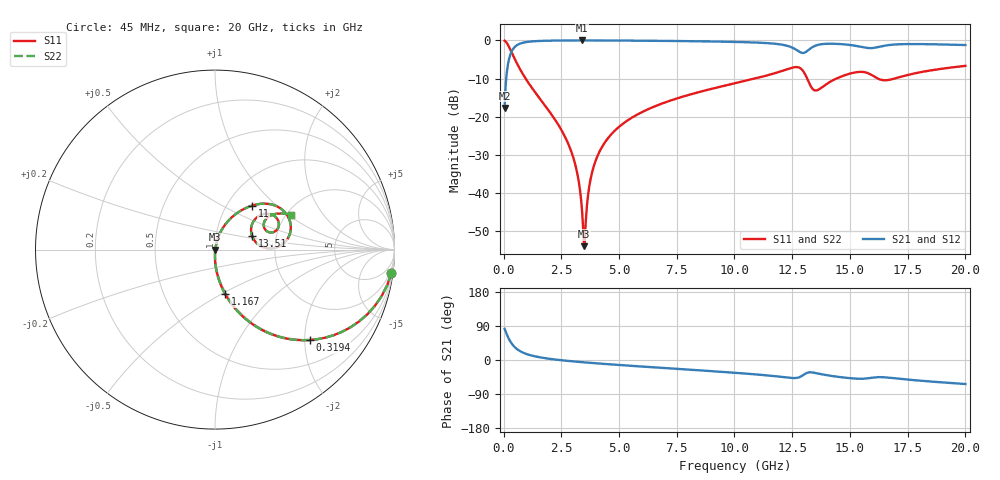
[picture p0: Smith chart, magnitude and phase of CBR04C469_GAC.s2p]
! S-parameter model data by Modelithics Inc.  support@modelithics.com 813-866-6335  Tampa FL USA
! S-Parameter data specifications:
! Substrate: 20-mil Rogers 4350B, substrate thickness, H=0.508mm, Dielectric constant, Er=3.75
! PCB Mounting Pad Footprint: Pad width, PadW=0.52mm , Pad length, PadL=0.52mm , Pad gap, PadG (edge-to-edge)=0.28mm , Reference planes=1.32mm apart
#  GHz  S  MA  R 50
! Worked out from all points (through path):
!   801 points, 45 MHz to 20 GHz, reference 50 ohm
!   highest |S21| = -0.02 dB at 3.412 GHz (marker M1); lowest = -17.7 dB at 45 MHz (marker M2)
!   group delay of S21, straight-line fit = 10.9 ps
!   lowest |S11| = -53.9 dB at 3.487 GHz (marker M3), VSWR 1.00, Z = 50.2 - j0.0601 ohm
!   |S11| at or under -10 dB: 954.2 MHz to 10.89 GHz (9.931 GHz wide, 168 % of centre); 13.15 GHz to 14.42 GHz (1.269 GHz wide, 9.21 % of centre); 16.21 GHz to 16.93 GHz (727.2 MHz wide, 4.39 % of centre)
!   |S22| runs from -53.9 to -0.1 dB; largest |S21 - S12| = 0
!   S11 on the Smith chart (normalised r, x): 45 MHz: 1, -15; 319.4 MHz: 0.98, -2.11; 1.167 GHz: 0.98, -0.52; 11 GHz: 1.31, +0.72; 13.51 GHz: 1.50, +0.24; 20 GHz: 2.11, +1.04
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0.045  0.9915 -7.5  0.1298 82.5  0.1298 82.5  0.9915 -7.5
0.194662  0.8694 -29.9  0.4939 60.0  0.4939 60.0  0.8694 -29.9
0.319381  0.7295 -43.7  0.6835 46.3  0.6835 46.3  0.7295 -43.7
0.64365  0.4583 -63.8  0.8879 26.1  0.8879 26.1  0.4583 -63.8
1.167469  0.2531 -77.2  0.9662 12.6  0.9662 12.6  0.2531 -77.2
2.8387  0.04143 -90.2  0.9973 -2.7  0.9973 -2.7  0.04143 -90.2
3.187912  0.01832 -88.7  0.9978 -4.6  0.9978 -4.6  0.01832 -88.7
3.387462  0.006456 -78.2  0.9979 -5.7  0.9979 -5.7  0.006456 -78.2
3.412406  0.005087 -73.3  0.9979 -5.8  0.9979 -5.8  0.005087 -73.3
3.487237  0.002008 -17.3  0.9979 -6.2  0.9979 -6.2  0.002008 -17.3
3.83645  0.01877 75.8  0.9976 -7.9  0.9976 -7.9  0.01877 75.8
4.310381  0.04235 76.9  0.9968 -10.1  0.9968 -10.1  0.04235 76.9
5.2333  0.08359 74.2  0.9939 -14.1  0.9939 -14.1  0.08359 74.2
6.704981  0.1426 68.7  0.9867 -20.1  0.9867 -20.1  0.1426 68.7
10.0225  0.2743 54.9  0.9551 -33.8  0.9551 -33.8  0.2743 54.9
10.99531  0.3223 49.7  0.9352 -38.4  0.9352 -38.4  0.3223 49.7
12.74137  0.4451 19.3  0.732 -46.7  0.732 -46.7  0.4451 19.3
13.36496  0.2345 9.0  0.8124 -32.8  0.8124 -32.8  0.2345 9.0
13.51463  0.22 19.9  0.8549 -34.3  0.8549 -34.3  0.22 19.9
15.28563  0.3832 28.4  0.8444 -49.2  0.8444 -49.2  0.3832 28.4
16.68248  0.3034 26.5  0.8684 -46.6  0.8684 -46.6  0.3034 26.5
20  0.4636 24.7  0.8695 -63.4  0.8695 -63.4  0.4636 24.7
